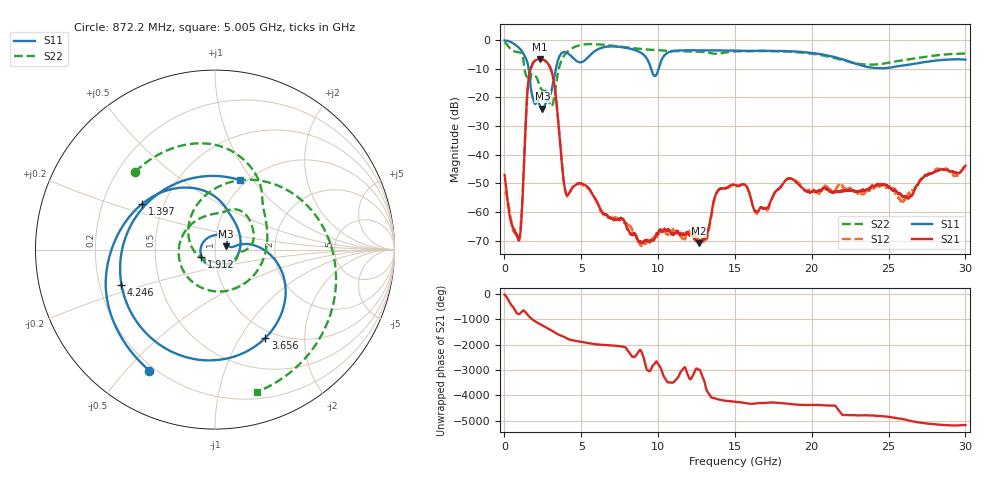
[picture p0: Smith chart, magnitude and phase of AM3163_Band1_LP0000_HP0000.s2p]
!Agilent Technologies,E8364B,MY43040894,A.07.50.67
!Agilent E8364B: A.07.50.67
!Date: Thursday, August 20, 2020 11:16:15
!Correction: S11(Full 2 Port(1,2))
!S21(Full 2 Port(1,2))
!S12(Full 2 Port(1,2))
!S22(Full 2 Port(1,2))
!S2P File: Measurements: S11, S21, S12, S22:
# Hz S  dB  R 50
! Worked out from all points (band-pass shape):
!   3201 points, 10 MHz to 30 GHz, reference 50 ohm
!   highest |S21| = -6.59 dB at 2.315 GHz (marker M1); lowest = -70.9 dB at 12.65 GHz (marker M2)
!   |S21| within 3 dB of the highest: 1.735 GHz to 2.98 GHz (1.245 GHz wide, 52.8 % of centre)
!   lowest |S11| = -23.9 dB at 2.465 GHz (marker M3), VSWR 1.14, Z = 56.5 + j2.14 ohm
!   |S11| at or under -10 dB: 1.578 GHz to 3.345 GHz (1.767 GHz wide, 71.8 % of centre); 9.545 GHz to 10.03 GHz (485.2 MHz wide, 4.96 % of centre)
!   |S22| runs from -23.2 to -0.7 dB; largest |S21 - S12| = 0.0052
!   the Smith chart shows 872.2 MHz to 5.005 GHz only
!   S11 on the Smith chart (normalised r, x): 872.2 MHz: 0.18, -0.58; 1.397 GHz: 0.38, +0.25; 1.912 GHz: 0.86, -0.07; 3.656 GHz: 0.89, -1.30; 4.246 GHz: 0.29, -0.17; 5.005 GHz: 0.94, +0.87
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1e7  -0.09 -8.7  -47.09 -21.9  -52.96 -53.8  -0.68 -29.4
4.504781e8  -0.74 -59.9  -64.07 -84.5  -63.41 -151.1  -3.37 -148.1
8.722125e8  -2.31 -118.5  -69.05 -59.4  -68.76 -34.7  -4.14 135.9
1.397038e9  -6.41 147.6  -27.26 -14.3  -27.31 -15.0  -12.07 -52.0
1.912491e9  -21.41 -152.3  -7.54 36.1  -7.54 36.1  -12.04 37.3
2.315481e9  -22.97 23.8  -6.59 -108.8  -6.59 -108.9  -16.27 -3.5
2.465431e9  -23.87 17.2  -6.73 -156.7  -6.73 -156.8  -17.55 -6.8
3.149578e9  -15.32 10.6  -12.67 -30.2  -12.69 -30.2  -22.23 -130.5
3.655659e9  -4.94 -60.3  -38.02 168.2  -38.03 169.7  -7.88 72.1
4.246088e9  -5.09 -159.4  -53.10 -0.4  -53.18 -1.6  -3.36 -8.6
5.005209e9  -7.71 69.8  -50.06 -86.1  -50.36 -87.0  -1.65 -73.5
5.014581e9  -7.70 68.1  -50.09 -87.0  -50.36 -87.9  -1.65 -74.2
5.679984e9  -4.71 -33.7  -53.32 -158.5  -53.46 -157.1  -1.36 -117.4
6.860841e9  -2.19 -137.7  -61.95 138.2  -62.01 136.1  -1.81 -177.5
8.55715e9  -3.56 127.3  -68.05 96.8  -68.77 10.8  -2.87 112.8
1.000979e10  -10.36 117.9  -67.36 113.3  -67.79 -137.0  -3.55 58.8
1.265266e10  -3.53 -1.7  -70.93 -98.3  -70.16 -19.1  -4.03 -30.9
1.5005e10  -3.65 -72.2  -50.59 68.4  -50.67 70.3  -3.92 -90.3
2.000958e10  -4.44 163.3  -52.87 -51.9  -51.88 -52.2  -4.71 136.8
2.275554e10  -8.04 60.3  -52.53 -98.4  -52.99 -100.8  -7.96 21.1
2.500479e10  -9.64 -62.0  -51.50 -163.4  -51.13 -163.6  -7.94 -91.6
3e10  -6.82 104.6  -43.89 -126.1  -44.37 -134.8  -4.67 102.4
